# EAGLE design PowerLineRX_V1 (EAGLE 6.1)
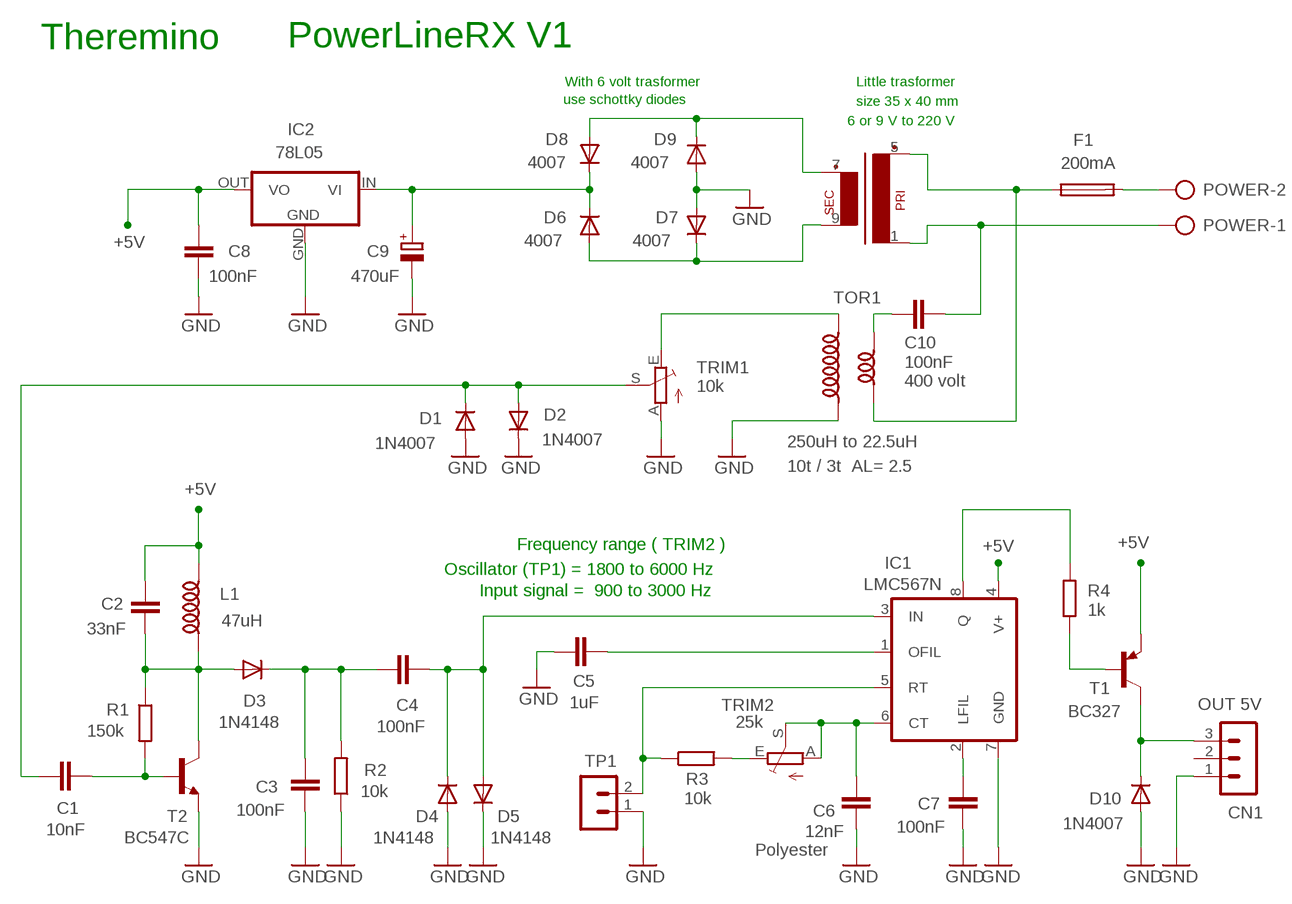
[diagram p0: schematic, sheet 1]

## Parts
C1  10nF  C5/2.5  [C5B2.5]
C2  33nF  C5/2.5  [C5B2.5]
C3  100nF  C5/2.5  [C5B2.5]
C4  100nF  C5/2.5  [C5B2.5]
C5  1uF  C7.5/3  [C7.5B3]
C6  12nF  C7.5/3  [C7.5B3]
C7  100nF  C7.5/3  [C7.5B3]
C8  100nF  C5/2.5  [C5B2.5]
C9  470uF  CPOL-EUE5-8.5  [E5-8,5]
C10  100nF  C10/4  [C10B4]
CN1  OUT 5V  MA03-1N  [MA03-1]
D1  1N4007  DIODE-DO35-10  [DO35-10]
D2  1N4007  DIODE-DO35-10  [DO35-10]
D3  1N4148  DIODE-DO35-10  [DO35-10]
D4  1N4148  DIODE-DO35-10  [DO35-10]
D5  1N4148  DIODE-DO35-10  [DO35-10]
D6  4007  DIODE-DO35-10  [DO35-10]
D7  4007  DIODE-DO35-10  [DO35-10]
D8  4007  DIODE-DO35-10  [DO35-10]
D9  4007  DIODE-DO35-10  [DO35-10]
D10  1N4007  DIODE-DO35-10  [DO35-10]
F1  200mA  FUSE_22,5  [FUSE_22,5]
IC1  LMC567N  LM567N  [DIL08]
IC2  78L05  78REG  [TO92-REG]
L1  47uH  INDUCTOR2250NH  [L250NH]
POWER  AK500/2  [AK500/2]
R1  150k  R-EU_0207/10  [0207/10]
R2  10k  R-EU_0207/10  [0207/10]
R3  10k  R-EU_0207/10  [0207/10]
R4  1k  R-EU_0207/10  [0207/10]
T1  BC327  -PNP-TO92-CBE  [TO92-CBE]
T2  BC547C  -NPN-TO92-CBE  [TO92-CBE]
TOR1  250uH to 22.5uH  INDUCTOR_DUALTOR2_REV2  [TOROID_2]
TP1  MA02-1N  [MA02-1]
TR1  EI38-1  [EI38-1]
TRIM1  10k  TRIMMERTRIM_2H  [TRIM_2H]
TRIM2  25k  TRIMMERTRIM_M1  [TRIM_M1]

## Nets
+5V: C2.1 C8.1 IC1.4(V+) IC2.OUT(VO) L1.2 T1.E
+7V: C9.V+ D6.C D8.C IC2.IN(VI)
GND: C3.2 C5.1 C6.1 C7.1 C8.2 C9.V- CN1.1 D1.A D2.C D4.A D5.C D7.A D9.A D10.A IC1.7(GND) IC2.GND R2.1 T2.E TOR1.2 TP1.1 TRIM1.A
N$1: C7.2 IC1.2(LFIL)
N$2: C10.2 POWER.1 TR1.1
N$3: C10.1 TOR1.4
N$5: C1.2 R1.2 T2.B
N$6: D8.A D9.C TR1.7(S3)
N$7: C2.2 D3.A L1.1 R1.1 T2.C
N$8: C3.1 C4.1 D3.C R2.2
N$9: F1.1 TOR1.3 TR1.5(P2)
N$10: F1.2 POWER.2
N$11: IC1.8(Q) R4.2
N$12: R4.1 T1.B
N$13: D6.A D7.C TR1.9(S4)
N$14: C5.2 IC1.1(OFIL)
N$15: C4.2 D4.C D5.A IC1.3(IN)
N$16: C6.2 IC1.6(CT) TRIM2.A TRIM2.S
N$17: IC1.5(RT) R3.1 TP1.2
N$18: R3.2 TRIM2.E
N$19: TOR1.1 TRIM1.E
N$20: CN1.3 D10.C T1.C
SIGNAL-IN: C1.1 D1.C D2.A TRIM1.S
Unconnected: CN1.2

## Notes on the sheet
- Theremino | PowerLineRX V1
- With 6 volt trasformer | Little trasformer
- use schottky diodes | size 35 x 40 mm
- 6 or 9 V to 220 V
- Frequency range ( TRIM2 )
- Oscillator (TP1) = 1800 to 6000 Hz
- Input signal =  900 to 3000 Hz

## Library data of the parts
C1-C4 C8 = 00-LIVIO:C: CAPACITOR
C5 C7 = capacitor-wima:C: CAPACITOR
C6 = capacitor-wima:C: CAPACITOR; 1: Polyester
C9 = 00-LIVIO:CPOL-EU: POLARIZED CAPACITOR, European symbol
C10 = 00-LIVIO:C: CAPACITOR; 1: 400 volt
CN1 = 03-con-lstb-M:MA03-1: PIN HEADER
D1-D10 = 00-LIVIO:DIODE-: DIODE
F1 = 00-LIVIO:FUSE_22,5: FUSE HOLDER
IC1 = linear:*567: TONE DECODER
IC2 = 00-LIVIO:78*: Positive VOLTAGE REGULATOR Source: http://cache.national.com/ds/LM/LM78L05.pdf http://www.fairchildsemi.com/ds/LM/LM7805.pdf
L1 = 00-LIVIO:INDUCTOR2: CHOKE
POWER = 07-con-ptr500:AK500/2: CONNECTOR
R1-R4 = 00-LIVIO:R-EU_: RESISTOR, European symbol
T1 = 00-LIVIO:*-PNP-: PNP Transistror
T2 = 00-LIVIO:*-NPN-: NPN Transistror
TOR1 = 00-LIVIO:INDUCTOR_DUAL; 1: 10t / 3t AL= 2.5
TP1 = 03-con-lstb-M:MA02-1: PIN HEADER
TR1 = trafo:EI38-1: TRANSFORMER 1 primary winding, 1 secondary winding ERA
TRIM1 TRIM2 = 00-LIVIO:TRIMMER: Horizzontal and Vertical trimmers

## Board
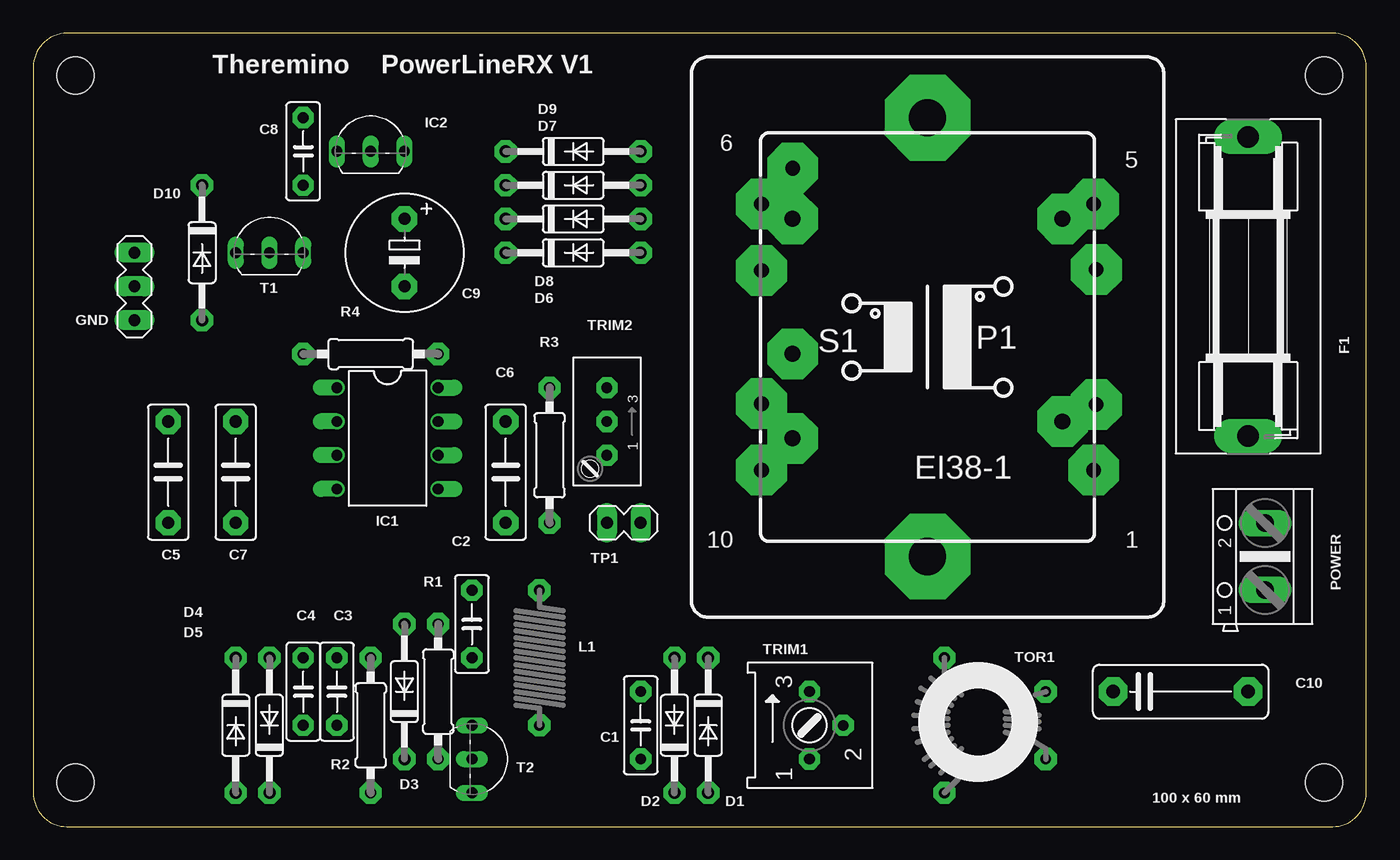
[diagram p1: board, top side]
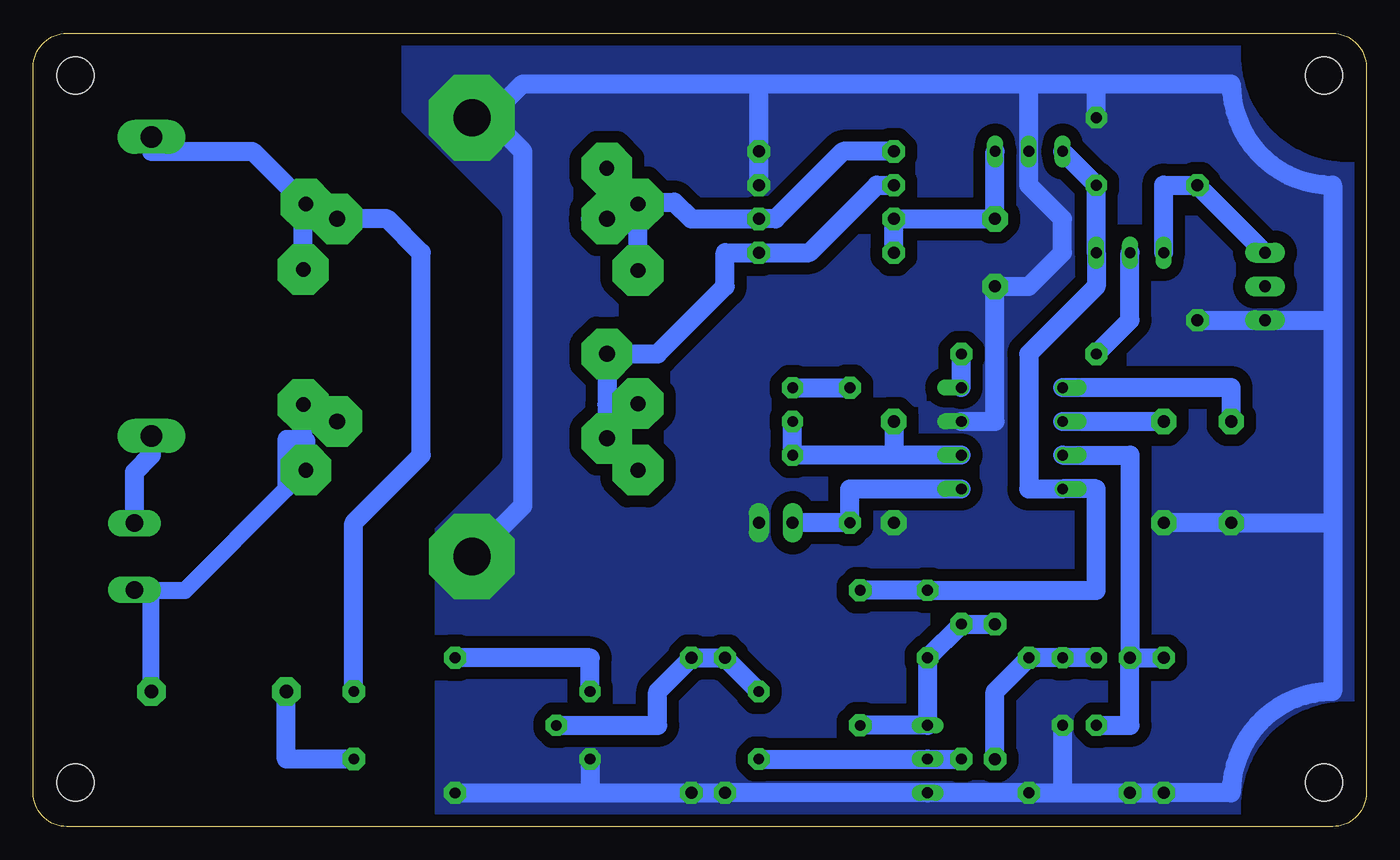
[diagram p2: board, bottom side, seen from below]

Size 100.33 x 59.69 mm. Coordinates in mm from the lower left corner, seen from the top.
Outline: 97.79,59.69 2.54,59.69 arc90 0,57.15 0,2.54 arc90 2.54,0 97.79,0 arc90 100.33,2.54 100.33,57.15 arc90 97.79,59.69
Copper layers (1*16): Top 0.035mm / dielectric 1.5mm / Bottom 0.035mm
Design rules: minimum track width 10mil, minimum drill 31mil, track to track 31mil, track to pad 31mil, pad to pad 31mil, via to via 31mil, smd to smd 31mil, copper to edge 31mil, drill to drill 8mil, minimum pad ring 5mil, minimum via ring 8mil, stop-mask expansion 4mil, vias tented up to drill 0mil, thermal gap 47mil
Holes 2.8 mm at 3.17,3.3 3.17,56.52 97.16,3.3 97.16,56.52
bRestrict: 8 lines

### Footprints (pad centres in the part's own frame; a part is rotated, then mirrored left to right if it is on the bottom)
C5B2.5 = drill 0.813 pad 1.6 octagon: 1 -2.54,0; 2 2.54,0
C7.5B3 = drill 0.914 pad 1.905 octagon: 1 -3.81,0; 2 3.81,0
E5-8,5 = drill 0.9 pad 1.93 octagon: V+ -2.54,0; V- 2.54,0
C10B4 = drill 1.016 pad 2.159 octagon: 1 -5.08,0; 2 5.08,0
MA03-1 = drill 0.9 pad 1.5 long: 1 -2.54,0; 2 0,0; 3 2.54,0
DO35-10 = drill 0.9 pad 1.676 octagon: A 5.08,0; C -5.08,0
FUSE_22,5 = drill 1.6 pad 2.54 long: 1 -11.252,0; 2 11.252,0
DIL08 = drill 0.813 offset: 1 -3.81,-3.81; 2 -1.27,-3.81; 3 1.27,-3.81; 4 3.81,-3.81; 5 3.81,3.81; 6 1.27,3.81; 7 -1.27,3.81; 8 -3.81,3.81
TO92-REG = drill 0.813 long: GND 0,0; IN 2.54,0; OUT -2.54,0
L250NH = drill 0.8 pad 1.676 octagon: 1 -5.08,0; 2 5.08,0
AK500/2 = drill 1.321 long: 1 -2.515,0; 2 2.515,0
0207/10 = drill 0.813 pad 1.676 octagon: 1 -5.08,0; 2 5.08,0
TO92-CBE = drill 0.813 long: B 0,0; C -2.54,0; E 2.54,0
TOROID_2 = drill 0.8 pad 1.676 octagon: 1 -2.54,5.08; 2 -2.54,-5.08; 3 5.08,2.54; 4 5.08,-2.54
MA02-1 = drill 0.9 pad 1.5 long: 1 -1.27,0; 2 1.27,0
EI38-1 = drill 1.118 pad 3.81 octagon: 1 -12.497,10.008; 5 -12.497,-10.008; 6 12.497,-10.008; 7 12.497,-5.004; 9 12.497,5.004; 10 12.497,10.008
TRIM_2H = drill 0.8 pad 1.6 octagon: A 2.54,0; E -2.54,0; S 0,2.54
TRIM_M1 = drill 0.8 pad 1.6 octagon: A 2.54,0; E -2.54,0; S 0,0

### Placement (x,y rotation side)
C1  45.72,7.62 270 top
C2  33.02,15.24 270 top
C3  22.86,10.16 270 top
C4  20.32,10.16 270 top
C5  10.16,26.67 90 top
C6  35.56,26.67 90 top
C7  15.24,26.67 90 top
C8  20.32,50.8 90 top
C9  27.94,43.18 270 top
C10  86.36,10.16 0 top
CN1  7.62,40.64 90 top
D1  50.8,7.62 270 top
D2  48.26,7.62 90 top
D3  27.94,10.16 90 top
D4  15.24,7.62 270 top
D5  17.78,7.62 90 top
D6  40.64,43.18 0 top
D7  40.64,48.26 0 top
D8  40.64,45.72 0 top
D9  40.64,50.8 0 top
D10  12.7,43.18 270 top
F1  91.44,40.64 270 top
IC1  26.67,29.21 270 top
IC2  25.4,50.8 0 top
L1  38.1,12.7 90 top
POWER  92.71,20.32 90 top
R1  30.48,10.16 270 top
R2  25.4,7.62 90 top
R3  38.86,27.94 90 top
R4  25.4,35.56 0 top
T1  17.78,43.18 0 top
T2  33.02,5.08 270 top
TOR1  71.12,7.62 0 top
TP1  44.45,22.86 180 top
TR1  67.31,36.83 180 top
TRIM1  58.42,7.62 270 top
TRIM2  43.18,30.48 270 top

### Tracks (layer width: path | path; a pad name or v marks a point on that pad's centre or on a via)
+5V
  Bottom 1.422: IC2.OUT C8.1 T1.E 20.32,40.64 25.4,35.56 25.4,25.4 IC1.4 20.32,25.4 20.32,17.78 C2.1 L1.2
+7V
  Bottom 1.422: IC2.IN C9.V+ D8.C D6.C
GND  (via drill 2.8 pad 6.45)
  Bottom 1.422: TRIM1.A 58.42,2.54 | 58.42,2.54 D1.A D2.C T2.E R2.1 22.86,2.54 | 22.86,2.54 D5.C D4.A 10.16,2.54 arc90 2.54,10.16 2.54,22.86 | C3.2 22.86,2.54 | TOR1.2 58.42,2.54 | v67.31,53.34 66.04,53.34 | v67.31,20.32 63.5,24.13 63.5,50.8 66.04,53.34 | 66.04,53.34 63.5,55.88 45.72,55.88 | 45.72,55.88 25.4,55.88 | 25.4,55.88 20.32,55.88 | 20.32,55.88 10.16,55.88 arc-90 2.54,48.26 2.54,38.1 | 2.54,38.1 2.54,22.86 | C8.2 20.32,55.88 | 25.4,55.88 IC2.GND 25.4,48.26 22.86,45.72 22.86,43.18 25.4,40.64 C9.V- 27.94,30.48 IC1.7 | D7.A D9.A 45.72,55.88 | CN1.1 D10.A 2.54,38.1 | 2.54,22.86 C5.1 C7.1
  pour Bottom (isolate 0.9, no thermals): -1,-1 101.33,-1 101.33,60.69 -1,60.69
N$1
  Bottom 1.422: IC1.2 C7.2
N$2  (via drill 1.1 pad 3.81, 1.2 pad 3.81)
  Bottom 1.27: C10.2 91.44,17.78 88.9,17.78 81.28,25.4 81.28,29.21 80.01,29.21
  Bottom 1.422: v77.47,30.48 80.01,30.48 | 80.01,30.48 v80.01,31.75 | TR1.1 79.81,29.01 80.01,29.21 80.01,30.48 | 91.44,17.78 92.73,17.78 POWER.1
N$3
  Bottom 1.422: TOR1.4 81.28,5.08 C10.1
N$5
  Bottom 1.422: C1.2 T2.B R1.2
N$6  (via drill 1.1 pad 3.81, 1.2 pad 3.81)
  Bottom 1.27: 57.15,46.86 57.05,46.97 57.28,46.97
  Bottom 1.422: TR1.7 54.81,46.79 54.61,46.99 | 54.61,46.99 57.15,46.99 | v57.15,45.72 57.15,46.99 | 57.15,46.99 v57.15,49.53 | 54.61,46.99 52.07,46.99 50.8,45.72 D8.A 44.45,45.72 39.37,50.8 D9.C | 57.15,46.99 58.42,45.72 55.88,45.72 55.88,45.8 57.05,46.97
N$7
  Bottom 1.422: L1.1 T2.C C2.2 R1.1 D3.A
N$8
  Bottom 1.422: D3.C 27.94,10.16 R2.2 C3.1 C4.1
N$9  (via drill 1.1 pad 3.81, 1.2 pad 3.81)
  Bottom 1.422: TOR1.3 76.2,22.86 71.12,27.94 71.12,43.18 73.66,45.72 v77.47,45.72 78.74,45.72 | v80.01,41.91 80.01,45.72 | 80.01,45.72 80.01,46.99 79.96,46.99 TR1.5 | 78.74,45.72 80.01,45.72 | F1.1 91.44,50.8 83.82,50.8 78.74,45.72
N$10
  Bottom 1.422: POWER.2 92.71,26.67 91.44,27.94 F1.2
N$11
  Bottom 1.422: IC1.8 R4.2
N$12
  Bottom 1.422: R4.1 17.78,38.1 T1.B
N$13  (via drill 1.2 pad 3.81)
  Bottom 1.422: 57.15,31.75 v57.15,35.56 53.34,35.56 48.26,40.64 48.26,43.18 D6.A 41.91,43.18 36.83,48.26 D7.C | 57.15,31.75 v57.15,29.21 | TR1.9 57.07,31.83 57.15,31.75
N$14
  Bottom 1.422: C5.2 10.16,33.02 IC1.1
N$15
  Bottom 1.422: C4.2 17.78,7.62 D5.A | D5.A D4.C | IC1.3 17.78,27.94 D5.A
N$16
  Bottom 1.422: IC1.6 35.56,27.94 | C6.2 35.56,27.94 | 35.56,27.94 TRIM2.A TRIM2.S
N$17
  Bottom 1.422: IC1.5 38.86,25.4 R3.1 TP1.2
N$18
  Bottom 1.422: TRIM2.E R3.2
N$19
  Bottom 1.422: TRIM1.E 58.42,12.7 TOR1.1
N$20
  Bottom 1.422: CN1.3 D10.C 15.24,48.26 T1.C
SIGNAL-IN
  Bottom 1.422: TRIM1.S 53.34,7.62 53.34,10.16 D1.C D2.A C1.1

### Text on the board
tNames: Theremino | PowerLineRX V1 | GND | 100 x 60 mm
